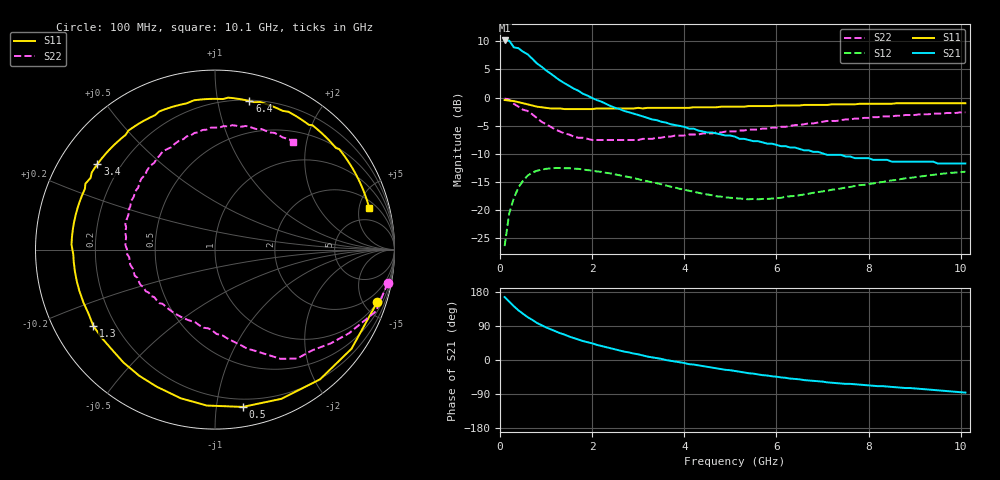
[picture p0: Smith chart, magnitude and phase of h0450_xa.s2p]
!HBFP-0450
!S and NOISE PARAMETERS at Vce=0.5V  Ic=1mA.  LAST UPDATED  09-04-98
# GHZ S MA R  50
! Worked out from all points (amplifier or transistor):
!   101 points, 100 MHz to 10.1 GHz, reference 50 ohm
!   highest |S21| = 10.1 dB at 100 MHz (marker M1)
!   |S21| within 3 dB of that: start of sweep to 669.3 MHz
!   unconditionally stable (mu >= 1): 3.291 GHz to end of sweep
!   at 1.7 GHz: K = 0.50, MSG = 6.9 dB, |S12| = -12.7 dB
!   at 5.1 GHz: K = 1.65, MAG = 0.7 dB, |S12| = -17.9 dB
!   at 10.1 GHz: K = 1.33, MAG = -2.7 dB, |S12| = -13.2 dB
!   lowest NFmin = 1.90 dB at 2 GHz
!   S11 on the Smith chart (normalised r, x): 100 MHz: 1.02, -6.15; 500 MHz: 0.14, -1.18; 1.3 GHz: 0.12, -0.28; 3.4 GHz: 0.12, +0.32; 6.4 GHz: 0.21, +1.24; 10.1 GHz: 2.86, +6.33
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0.1  0.95 -18.0  3.21 166.0  0.048 78.0  0.98 -11.0
0.2  0.94 -36.0  3.2 154.0  0.094 67.0  0.96 -21.0
0.3  0.93 -51.0  2.79 142.0  0.128 57.0  0.88 -32.0
0.4  0.91 -66.0  2.74 131.0  0.159 48.0  0.83 -39.0
0.5  0.89 -80.0  2.55 122.0  0.183 40.0  0.78 -46.0
0.6  0.87 -93.0  2.42 113.0  0.203 33.0  0.76 -53.0
0.8  0.83 -113.0  2.01 98.0  0.224 21.0  0.66 -63.0
1  0.81 -129.0  1.74 86.0  0.233 12.0  0.58 -72.0
1.3  0.8 -148.0  1.42 71.0  0.237 1.0  0.5 -82.0
1.5  0.79 -158.0  1.27 62.0  0.236 -5.0  0.47 -89.0
1.8  0.79 -171.0  1.08 50.0  0.23 -13.0  0.44 -98.0
2.5  0.8 166.0  0.81 28.0  0.208 -27.0  0.42 -119.0
3.4  0.81 144.0  0.63 5.0  0.174 -38.0  0.44 -144.0
3.5  0.81 141.0  0.61 3.0  0.17 -39.0  0.44 -147.0
4.1  0.81 128.0  0.53 -11.0  0.149 -42.0  0.47 -162.0
5.1  0.83 105.0  0.45 -29.0  0.128 -41.0  0.5 172.0
6.4  0.85 77.0  0.36 -50.0  0.134 -35.0  0.57 136.0
6.8  0.86 69.0  0.33 -55.0  0.143 -36.0  0.59 125.0
7.5  0.87 57.0  0.3 -63.0  0.159 -39.0  0.64 108.0
8.5  0.88 40.0  0.27 -71.0  0.184 -47.0  0.68 88.0
9.1  0.89 31.0  0.27 -76.0  0.199 -54.0  0.71 76.0
10.1  0.89 15.0  0.26 -86.0  0.22 -68.0  0.74 54.0
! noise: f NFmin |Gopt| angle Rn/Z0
1.8  2.07  0.67  157  0.1
2  1.9  0.73  166  0.05
2.5  2.37  0.74  -175  0.05
3.5  2.79  0.8  -146  0.32
4  3  0.84  -134  0.64
5  3.38  0.86  -110  1.83
5.5  3.59  0.9  -98  2.88
7  4.55  0.9  -67  6.65
8  4.63  0.9  -50  8.49
10  5.42  0.84  -18  9.79
